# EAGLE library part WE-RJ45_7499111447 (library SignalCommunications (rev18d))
Order Code 7499111447 Design THT xBase-T 10/100/1000 Base-T Ports 1x1 Application Standard Tab Position Up LED (Left-Right) GREEN/YELLOW-GREEN/YELLOW EMI Fingers yes Details see: http://katalog.we-online.de/en/pbs/WE-LAN_RJ45/7499111447? Updated by Yingchun Shan 2016-08-29 2016(C) Würth Elektronik
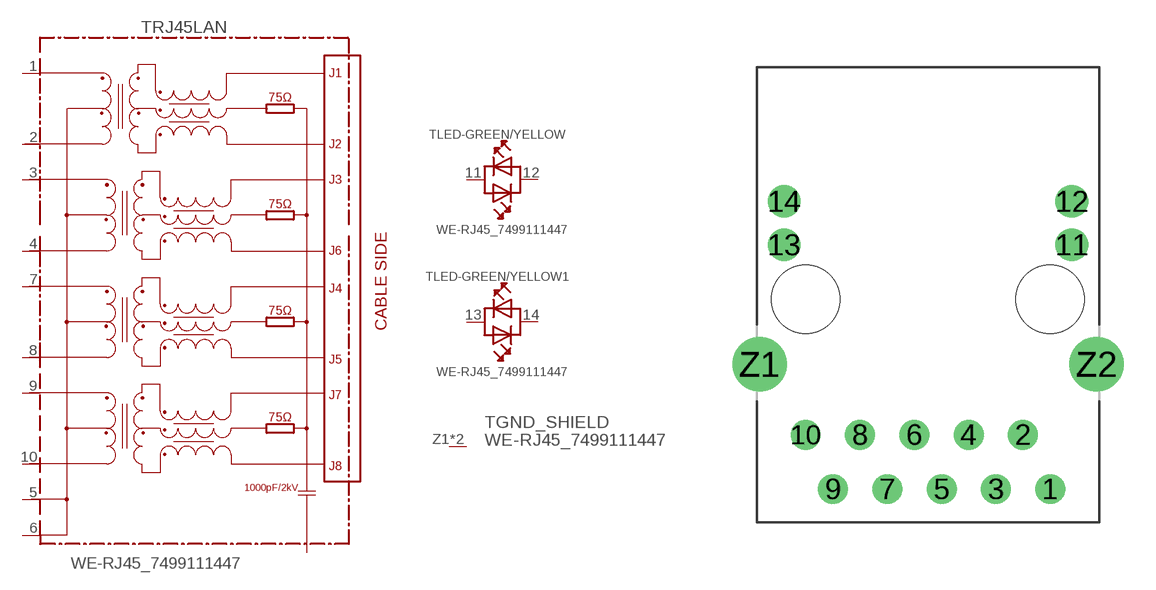
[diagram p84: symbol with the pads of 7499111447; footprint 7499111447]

Designator prefix T; gates RJ45LAN=7499111447 LED-GREEN/YELLOW=LED-DUAL-1 LED-GREEN/YELLOW1=LED-DUAL-1 GND_SHIELD=GNDPIN

## WE-RJ45_7499111447 (COMPANY-URL: http://www.we-online.de; CREATED-BY: Christin Zierenner; CREATED-DATE: AUG 2012; DATASHEET-URL: http://katalog.we-online.de/kataloge/eisos/media/pdf/7499111447.pdf; MANUFACTURER: Würth Elektronik eiSos GmbH)  [7499111447]
1  RJ45LAN:1
2  RJ45LAN:2
3  RJ45LAN:3
4  RJ45LAN:4
5  RJ45LAN:5
6  RJ45LAN:6
7  RJ45LAN:7
8  RJ45LAN:8
9  RJ45LAN:9
10  RJ45LAN:10
11  LED-GREEN/YELLOW:AK1  pas
12  LED-GREEN/YELLOW:AK2  pas
13  LED-GREEN/YELLOW1:AK1  pas
14  LED-GREEN/YELLOW1:AK2  pas
Z1  GND_SHIELD:GND  pwr
Z2  GND_SHIELD:GND  pwr

## Footprint 7499111447 (pad centres in mm)
MAX HEIGHT=13.55mm PORTS----1X1 LED -YES
drill 0.89: 1 5.72,-8.89; 2 4.44,-6.35; 3 3.18,-8.89; 4 1.9,-6.35; 5 0.64,-8.89; 6 -0.64,-6.35; 7 -1.9,-8.89; 8 -3.18,-6.35; 9 -4.44,-8.89; 10 -5.72,-6.35
drill 1.02: 11 6.725,2.54; 12 6.725,4.57; 13 -6.725,2.54; 14 -6.725,4.57
drill 1.7: Z1 -7.875,-3.05; Z2 7.875,-3.05
hole 3.2 at 5.715,0
hole 3.2 at -5.715,0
